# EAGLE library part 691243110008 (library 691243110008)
WR-TBL Series 2431 - 3.50 mm Horizontal cable entry with rising clamp 8 Way PCB Terminal Block Source: Datasheet
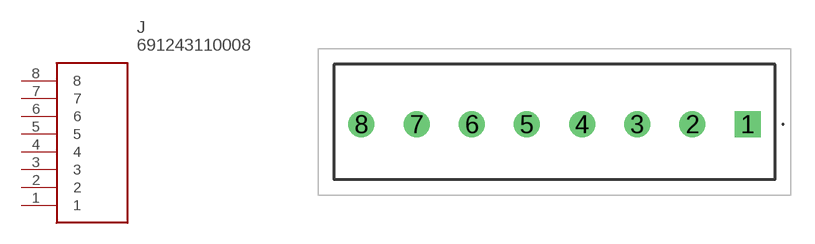
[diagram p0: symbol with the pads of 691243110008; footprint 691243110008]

Designator prefix J

## 691243110008 (Description: WR-TBL Series 2431 - 3.50 mm Horizontal cable entry with rising clamp 8 Way PCB Terminal Block; Height: 9.2mm; Manufacturer_Name: Wurth Elektronik; Manufacturer_Part_Number: 691243110008; Mouser_Part_Number: 710-691243110008; Mouser_Price-Stock: https://www.mouser.co.uk/ProductDetail/Wurth-Elektronik/691243110008?qs=sPbYRqrBIVmY2d1lpdr8tw%3D%3D)  [691243110008]
1  1
2  2
3  3
4  4
5  5
6  6
7  7
8  8

## Footprint 691243110008 (pad centres in mm)
691243110008-3
drill 1.1 pad 1.65 square: 1 0,0
drill 1.1 pad 1.65: 2 -3.5,0; 3 -7,0; 4 -10.5,0; 5 -14,0; 6 -17.5,0; 7 -21,0; 8 -24.5,0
